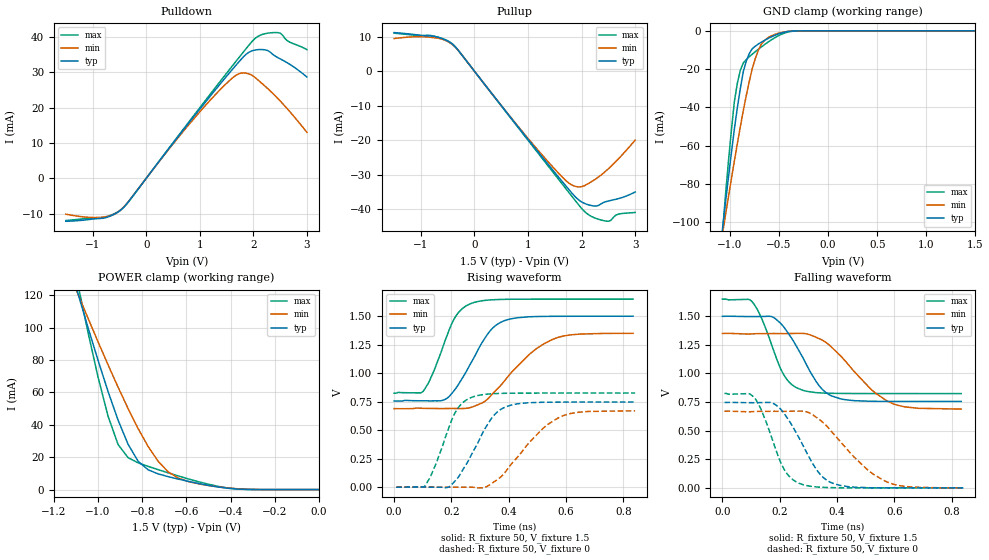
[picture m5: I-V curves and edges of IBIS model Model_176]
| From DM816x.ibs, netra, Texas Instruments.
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| Model based on original model for BSHTLTCSCDDVGPBFZ
|   Sub model FAST_8MA_10PER_P_1P5
[model]   Model_176
|[Description]  1.5V-3-STATE-X-FAST, 8MA, +-10%
|[Input Load]
|[Output Drive] FAST, 8MA
|Voltage   1.5V
|Mode   3-STATE
Model_type   3-state
Polarity   Non-Inverting
Enable   Active-Low
Cref =  15.0000pF
Rref =  100.0000M
Vref =  0V
Vmeas =  0.75
C_comp   1.5249p   1.4275p   1.6205p
[Model Spec]
[Temperature Range]   25   125   -40
[Voltage Range]   1.5   1.35   1.65
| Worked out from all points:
|   slope of the pulldown table from 0 to 0.225 V, typ, clamps not added: 50.1 ohm
|   slope of the pullup table from 0 to 0.225 V, typ, clamps not added: 50.1 ohm
|   GND clamp passes 1 mA (typ) near -0.47 V on its own axis
|   POWER clamp passes 1 mA (typ) near -0.42 V on its own axis
|   rising waveform, R_fixture 50, V_fixture 1.5: 20-80 % time 103ps typ, 154ps min, 78.2ps max; typ from 0.756 V to 1.5 V
|   rising waveform, R_fixture 50, V_fixture 0: 20-80 % time 99.2ps typ, 141ps min, 75.3ps max; typ from 0 V to 0.747 V
|   falling waveform, R_fixture 50, V_fixture 1.5: 20-80 % time 104ps typ, 152ps min, 77.8ps max; typ from 1.5 V to 0.755 V
|   falling waveform, R_fixture 50, V_fixture 0: 20-80 % time 101ps typ, 153ps min, 75.6ps max; typ from 0.746 V to 0 V
[POWER_clamp]
-1.5V     321.6mA    260.6mA    415.8mA
-1.091V   121.1mA    120.8mA    126.6mA
-1.076V   114.1mA    115.8mA    116.8mA
-1V       79.88mA    91.3mA     69.56mA
-954.5mV  60.58mA    77.05mA    45.34mA
-909.1mV  42.84mA    63.2mA     27.8mA
-818.2mV  17.47mA    37.6mA     16.51mA
-772.7mV  12.19mA    26.53mA    14.33mA
-681.8mV  7.985mA    10.89mA    10.33mA
-590.9mV  5.092mA    4.952mA    6.596mA
-363.6mV  298.9uA    465.6uA    298.1uA
0V        1.518nA    23.05nA    396.5pA
[Pulldown]
-1.5V     -12.15mA   -10.14mA   -11.93mA
-772.7mV  -11.18mA   -10.9mA    -10.98mA
-590.9mV  -10.12mA   -10.11mA   -9.968mA
-409.1mV  -8.017mA   -7.951mA   -8.019mA
954.5mV   18.69mA    17.99mA    19.06mA
1.455V    28.01mA    26.18mA    28.82mA
1.727V    32.86mA    29.54mA    34.05mA
2V        36.15mA    28.87mA    39.08mA
2.318V    35.62mA    24.67mA    41.12mA
2.5V      33.77mA    21.88mA    41.05mA
2.636V    32.63mA    19.61mA    38.86mA
3V        28.64mA    13.01mA    36.37mA
[Pullup]
-1.5V     11.21mA    9.48mA     11.04mA
-772.7mV  10.17mA    9.762mA    10.21mA
-409.1mV  7.827mA    7.7mA      7.892mA
1.227V    -24.14mA   -23.61mA   -24.51mA
1.682V    -32.78mA   -31.32mA   -33.54mA
1.864V    -36.09mA   -33.28mA   -37.13mA
2V        -37.87mA   -33.46mA   -39.75mA
2.182V    -38.93mA   -32.03mA   -42.07mA
2.409V    -38.05mA   -29.51mA   -43.28mA
2.545V    -37.45mA   -27.6mA    -43.23mA
2.682V    -36.95mA   -25.48mA   -41.44mA
3V        -34.98mA   -19.98mA   -40.92mA
[GND_clamp]
-1.5V     -310mA     -250.5mA   -402.4mA
-1.076V   -103.5mA   -106.1mA   -105.2mA
-1.045V   -89.74mA   -96.32mA   -85.93mA
-954.5mV  -51.19mA   -67.85mA   -36.85mA
-924.2mV  -40.06mA   -58.84mA   -27.27mA
-863.6mV  -21.23mA   -41.55mA   -16.73mA
-833.3mV  -15.79mA   -33.74mA   -15.03mA
-772.7mV  -9.342mA   -19.74mA   -12.19mA
-712.1mV  -6.927mA   -10.35mA   -9.702mA
-621.2mV  -4.26mA    -3.894mA   -6.224mA
-409.1mV  -336.9uA   -288.9uA   -618.6uA
1.5V      1.518nA    2.298uA    269.6pA
[Ramp]
dV/dt_f   0.595968/0.15569478n   0.5294/0.22543131n   0.660776/0.12038263n
dV/dt_r  0.6013656/0.14771921n 0.54143776/0.21236034n 0.66243504/0.11603173n
R_load = 50
[Rising Waveform]
R_fixture = 50
V_fixture = 1.5
V_fixture_min = 1.35
V_fixture_max = 1.65
0s        755.8mV    689.4mV    824.8mV
101.5ps   757.9mV    691.8mV    842.2mV
187.9ps   786.7mV    690.7mV    1.352V
220ps     884.4mV    690.1mV    1.518V
264.4ps   1.074V     697.3mV    1.608V
334.6ps   1.371V     795.6mV    1.643V
399.8ps   1.473V     978.9mV    1.649V
494.4ps   1.497V     1.212V     1.65V
567.1ps   1.499V     1.311V     1.65V
833.3ps   1.5V       1.35V      1.65V
[Rising Waveform]
R_fixture = 50
V_fixture = 0
V_fixture_min = 0
V_fixture_max = 0
7.45ps    0V         0V         0V
107.2ps   2.708mV    2.692mV    11.81mV
193.3ps   5.483mV    0V         537.6mV
227.2ps   100.1mV    0V         708.8mV
274.3ps   307.5mV    0V         792.1mV
343.4ps   616.3mV    38.03mV    820.1mV
405ps     717.8mV    190.4mV    824.5mV
517.3ps   745.1mV    510.8mV    825.8mV
584.3ps   746.6mV    622.1mV    825.9mV
840.8ps   747.2mV    670.5mV    826mV
[Falling Waveform]
R_fixture = 50
V_fixture = 1.5
V_fixture_min = 1.35
V_fixture_max = 1.65
0s        1.499V     1.35V      1.649V
105.5ps   1.497V     1.346V     1.622V
173.5ps   1.495V     1.349V     1.239V
212.6ps   1.411V     1.348V     995.6mV
279.3ps   1.145V     1.35V      853.9mV
342.9ps   876.7mV    1.298V     829.8mV
413.7ps   776.8mV    1.15V      825.1mV
520.8ps   756.8mV    856.7mV    824.3mV
596.6ps   755.4mV    734mV      824.2mV
833.3ps   755.1mV    688.5mV    824.1mV
[Falling Waveform]
R_fixture = 50
V_fixture = 0
V_fixture_min = 0
V_fixture_max = 0
7.45ps    746.2mV    669.6mV    825.4mV
113.5ps   743.9mV    667.4mV    783.5mV
173.5ps   742.3mV    669.2mV    429.6mV
212.5ps   659.9mV    668.6mV    175.7mV
266.4ps   441.8mV    671mV      41.12mV
339.8ps   122.3mV    594.1mV    6.189mV
407.4ps   22.79mV    416.3mV    0V
507.2ps   2.34mV     156.4mV    0V
584.2ps   0V         41.78mV    0V
840.8ps   0V         0V         0V
